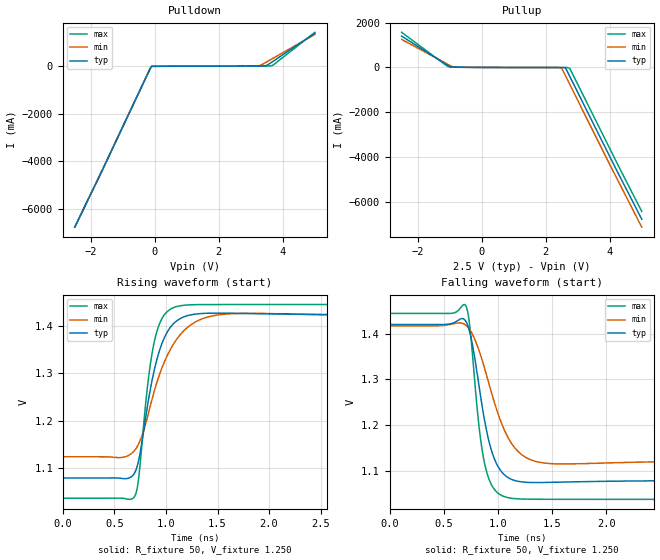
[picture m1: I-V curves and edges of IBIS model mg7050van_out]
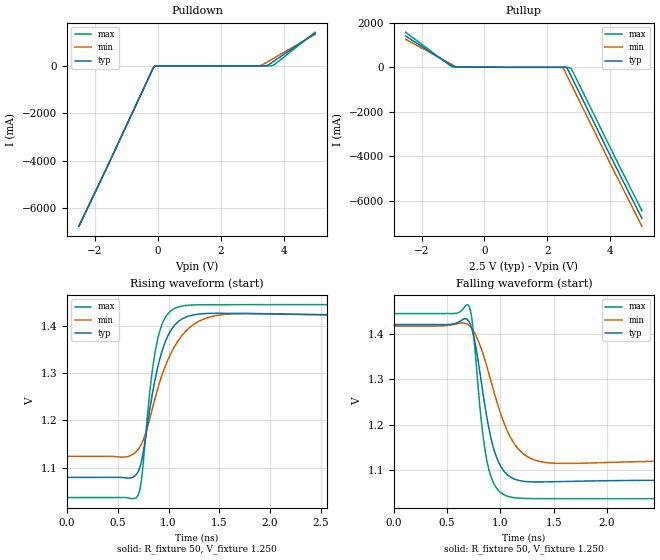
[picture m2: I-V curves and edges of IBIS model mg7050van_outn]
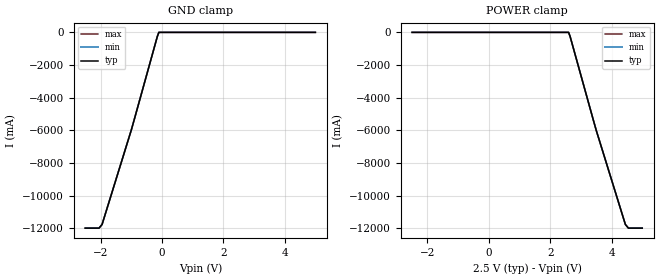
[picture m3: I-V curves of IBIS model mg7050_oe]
|   IBIS File mg7050van_4out_25v.ibs
[IBIS Ver]   3.2
[Comment Char]   |_char
[File name]   mg7050van_4out_25v.ibs
[File Rev]   1.0
[Date]   Aug 02, 2013
[Source]
|   Component MG7050VAN LVDS 4-OUTPUT 2.5V
[Component]   mg7050van-lvds-4out
[Manufacturer]   Seiko Epson Corporation
[Package]
| variable   typ   min   max
R_pkg   0.27   NA   NA
L_pkg   1.66n   NA   NA
C_pkg   0.53p   NA   NA
[Pin]   signal_name   model_name   R_pin   L_pin   C_pin
1   vcc1   POWER   NA   NA   NA
2   out1p   mg7050van_out   0.34   2.1nH   0.58pF
3   out1n   mg7050van_outn  0.25   1.5nH   0.50pF
4   out2p   mg7050van_out   0.22   1.3nH   0.44pF
5   out2n   mg7050van_outn  0.25   1.7nH   0.59pF
6   fsel   mg7050_fsel   NA   NA   NA
7   oe   mg7050_oe   NA   NA   NA
8   out3n   mg7050van_outn  0.25   1.7nH   0.62pF
9   out3p   mg7050van_out   0.22   1.3nH   0.49pF
10   out4n   mg7050van_outn  0.25   1.5nH   0.46pF
11   out4p   mg7050van_out   0.34   2.1nH   0.57pF
12   vcc2   POWER   NA   NA   NA
13   vcc   POWER   NA   NA   NA
14   gnd   GND   NA   NA   NA
[Diff Pin] inv_pin vdiff   tdelay_typ
2   3   0   0
4   5   0   0
9   8   0   0
11   10   0   0
| Models and submodels in the file (4): mg7050van_out (Output), mg7050van_outn (Output), mg7050_oe (Input), mg7050_fsel (Input)
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[Model]   mg7050van_out
Model_type Output
Enable Active-High
Polarity Non-Inverting
Vref=1.250
Vmeas=1.250
Rref=50
Cref=0
C_comp   0.12p   0.12p   0.12p
[Temperature Range] 25   90   -40
[Voltage Range]   2.5   2.375   2.625
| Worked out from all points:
|   slope of the pulldown table from 0 to 0.375 V, typ, clamps not added: 217 ohm
|   slope of the pullup table from 0 to 0.375 V, typ, clamps not added: 163 ohm
|   falling waveform, R_fixture 50, V_fixture 1.250: 20-80 % time 155ps typ, 241ps min, 113ps max; typ from 1.42 V to 1.08 V
|   rising waveform, R_fixture 50, V_fixture 1.250: 20-80 % time 186ps typ, 282ps min, 130ps max; typ from 1.08 V to 1.42 V
[Pullup]
-2.5V     1.396A     1.249A     1.566A
-1.15V    170.5mA    209.4mA    134.2mA
-1V       37.94mA    93.89mA    18.04mA
-900mV    10.86mA    25.98mA    12.65mA
-750mV    7.276mA    5.564mA    10.29mA
2.4V      -3.756mA   -3.229mA   -4.673mA
2.5V      -3.763mA   -40.87mA   -4.686mA
2.6V      -3.771mA   -323.5mA   -4.697mA
2.65V     -108.9mA   -466.8mA   -4.702mA
2.75V     -395.4mA   -753.3mA   -41.59mA
4.15V     -4.407A    -4.755A    -4.05A
5V        -6.777A    -7.132A    -6.431A
[Pulldown]
-2.5V     -6.778A    -6.782A    -6.778A
-1.65V    -4.407A    -4.406A    -4.408A
-150mV    -107.9mA   -107.7mA   -108mA
-100mV    -862.3uA   -635.9uA   -1.116mA
3.2V      7.339mA    9.603mA    9.752mA
3.35V     8.844mA    74.73mA    11.24mA
3.5V      37.82mA    190mA      12.9mA
3.65V     170.3mA    305.3mA    24.11mA
5V        1.394A     1.344A     1.433A
[Falling Waveform]
R_fixture=50
V_fixture=1.250
V_fixture_min=1.271
V_fixture_max=1.238
0s        1.42V      1.417V     1.444V
700ps     1.429V     1.419V     1.463V
740ps     1.403V     1.409V     1.417V
820ps     1.295V     1.367V     1.209V
870ps     1.219V     1.33V      1.124V
950ps     1.137V     1.264V     1.065V
1.04ns    1.096V     1.2V       1.045V
1.2ns     1.076V     1.139V     1.038V
1.44ns    1.074V     1.116V     1.037V
4ns       1.078V     1.123V     1.037V
[Rising Waveform]
R_fixture=50
V_fixture=1.250
V_fixture_min=1.271
V_fixture_max=1.238
0s        1.08V      1.124V     1.037V
700ps     1.092V     1.138V     1.042V
730ps     1.111V     1.149V     1.069V
820ps     1.23V      1.207V     1.27V
880ps     1.3V       1.257V     1.359V
950ps     1.356V     1.305V     1.41V
1.06ns    1.401V     1.357V     1.437V
1.26ns    1.424V     1.405V     1.444V
1.56ns    1.426V     1.424V     1.445V
4ns       1.423V     1.42V      1.445V
[Ramp]
R_load=50
dV/dt_r   2.065E-1/1.861E-10   1.775E-1/2.817E-10   2.447E-1/1.298E-10
dV/dt_f   2.054E-1/1.553E-10   1.766E-1/2.411E-10   2.444E-1/1.127E-10
|[End   mg7050van_out
[Model]   mg7050van_outn
Model_type Output
Enable Active-High
Polarity Inverting
Vref=1.250
Vmeas=1.250
Rref=50
Cref=0
C_comp   0.12p   0.12p   0.12p
[Temperature Range] 25   90   -40
[Voltage Range]   2.5   2.375   2.625
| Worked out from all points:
|   slope of the pulldown table from 0 to 0.375 V, typ, clamps not added: 217 ohm
|   slope of the pullup table from 0 to 0.375 V, typ, clamps not added: 163 ohm
|   falling waveform, R_fixture 50, V_fixture 1.250: 20-80 % time 155ps typ, 241ps min, 113ps max; typ from 1.42 V to 1.08 V
|   rising waveform, R_fixture 50, V_fixture 1.250: 20-80 % time 186ps typ, 282ps min, 130ps max; typ from 1.08 V to 1.42 V
[Pullup]
-2.5V     1.396A     1.249A     1.566A
-1.15V    170.5mA    209.4mA    134.2mA
-1V       37.94mA    93.89mA    18.04mA
-900mV    10.86mA    25.98mA    12.65mA
-750mV    7.276mA    5.564mA    10.29mA
2.4V      -3.756mA   -3.229mA   -4.673mA
2.5V      -3.763mA   -40.87mA   -4.686mA
2.6V      -3.771mA   -323.5mA   -4.697mA
2.65V     -108.9mA   -466.8mA   -4.702mA
2.75V     -395.4mA   -753.3mA   -41.59mA
4.15V     -4.407A    -4.755A    -4.05A
5V        -6.777A    -7.132A    -6.431A
[Pulldown]
-2.5V     -6.778A    -6.782A    -6.778A
-1.65V    -4.407A    -4.406A    -4.408A
-150mV    -107.9mA   -107.7mA   -108mA
-100mV    -862.3uA   -635.9uA   -1.116mA
3.2V      7.339mA    9.603mA    9.752mA
3.35V     8.844mA    74.73mA    11.24mA
3.5V      37.82mA    190mA      12.9mA
3.65V     170.3mA    305.3mA    24.11mA
5V        1.394A     1.344A     1.433A
[Falling Waveform]
R_fixture=50
V_fixture=1.250
V_fixture_min=1.271
V_fixture_max=1.238
0s        1.42V      1.417V     1.444V
700ps     1.429V     1.419V     1.463V
740ps     1.403V     1.409V     1.417V
820ps     1.295V     1.367V     1.209V
870ps     1.219V     1.33V      1.124V
950ps     1.137V     1.264V     1.065V
1.04ns    1.096V     1.2V       1.045V
1.2ns     1.076V     1.139V     1.038V
1.44ns    1.074V     1.116V     1.037V
4ns       1.078V     1.123V     1.037V
[Rising Waveform]
R_fixture=50
V_fixture=1.250
V_fixture_min=1.271
V_fixture_max=1.238
0s        1.08V      1.124V     1.037V
700ps     1.092V     1.138V     1.042V
730ps     1.111V     1.149V     1.069V
820ps     1.23V      1.207V     1.27V
880ps     1.3V       1.257V     1.359V
950ps     1.356V     1.305V     1.41V
1.06ns    1.401V     1.357V     1.437V
1.26ns    1.424V     1.405V     1.444V
1.56ns    1.426V     1.424V     1.445V
4ns       1.423V     1.42V      1.445V
[Ramp]
R_load=50
dV/dt_r   2.065E-1/1.861E-10   1.775E-1/2.817E-10   2.447E-1/1.298E-10
dV/dt_f   2.054E-1/1.553E-10   1.766E-1/2.411E-10   2.444E-1/1.127E-10
|[End   mg7050van_outn
[Model]   mg7050_oe
Model_type Input
Vinh=1.75
Vinl=0.75
C_comp   3p   3p   3p
[Temperature Range] 25   90   -40
[Voltage Range]   2.5   2.375   2.625
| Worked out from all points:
|   GND clamp passes 1 mA (typ) near -0.10 V on its own axis
[GND Clamp]
-2.5V     -12A       -12A       -12A
-2.05V    -12A       -12A       -12A
-1.95V    -11.77A    -11.77A    -11.77A
-1V       -6A        -6A        -6A
-150mV    -254mA     -254mA     -254mA
-100mV    -25.23uA   -22.27uA   -29.37uA
5V        24.28uA    23.68uA    25.61uA
[POWER Clamp]
-2.5V     24.28uA    23.68uA    25.61uA
2.6V      -25.23uA   -22.27uA   -29.37uA
2.65V     -254mA     -254mA     -254mA
3.5V      -6A        -6A        -6A
4.45V     -11.77A    -11.77A    -11.77A
4.55V     -12A       -12A       -12A
5V        -12A       -12A       -12A
